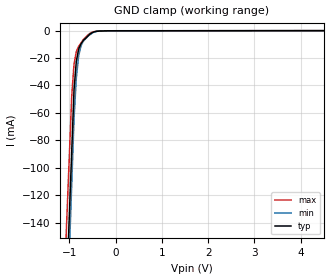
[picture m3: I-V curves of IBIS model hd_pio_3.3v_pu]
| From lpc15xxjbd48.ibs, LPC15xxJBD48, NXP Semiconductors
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[Model] hd_pio_3.3v_pu
Model_type Input
Vinl = 990.000mV
Vinh = 2.31000V
C_comp 598.000fF 598.000fF 598.000fF
| variable typ   min   max
[Voltage Range] 3.30000V 3.00000V 3.60000V
[POWER Clamp Reference] 3.30000V 3.00000V 3.60000V
[GND Clamp Reference] 0.00000V 0.00000V 0.00000V
[Temperature Range]   25   85   -40
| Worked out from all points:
|   GND clamp passes 1 mA (typ) near -0.47 V on its own axis
[GND Clamp]
-3.3V     -2.207A    -2.368A    -2.028A
-950mV    -88.27mA   -112.1mA   -48mA
-900mV    -43.2mA    -64.15mA   -24.39mA
-850mV    -22.27mA   -34.35mA   -15.18mA
-800mV    -13.45mA   -18.38mA   -11.42mA
-750mV    -9.601mA   -11.14mA   -8.989mA
-700mV    -7.175mA   -7.813mA   -6.557mA
-600mV    -3.919mA   -4.087mA   -3.117mA
-500mV    -1.3mA     -1.593mA   -1.015mA
-350mV    -283.3uA   -296.8uA   -262.2uA
319.2uV   -107.9uA   -62.22uA   -80.97uA
6.6V      60.08uA    42.87uA    37.81uA
[POWER Clamp]
-3.3V     0A         0A         0A
6.6V      0A         0A         0A
